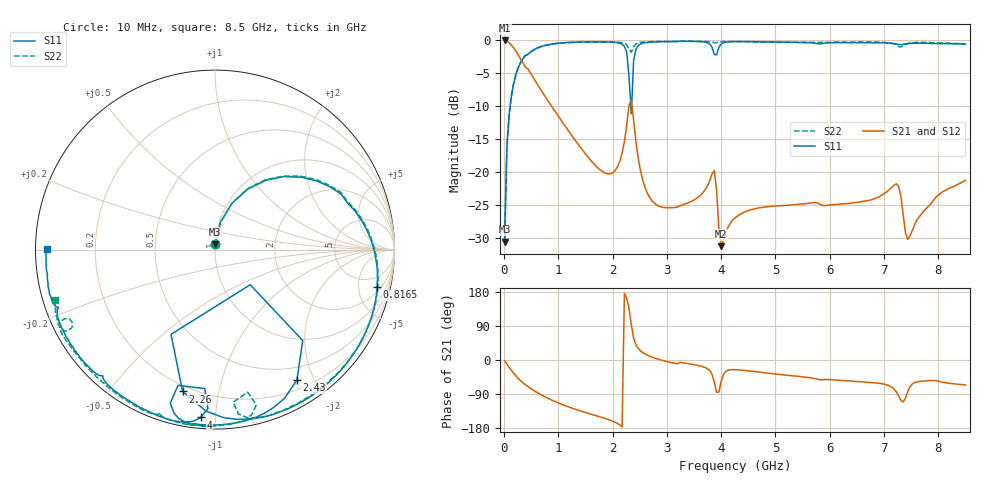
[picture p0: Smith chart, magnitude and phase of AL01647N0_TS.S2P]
!AVX CORPORATION
!PART NUMBER AL01647N0_TS
!DESCRIPTION: AIR CORE INDUCTOR, 47nH, 6 TURNS
!Agilent Technologies,E5071C,MY46102230,A.09.54
!Date: Mon Sep 03 16:36:54 2012
!Data & Calibration Information:
!Freq	S11:SOLT2(ON)	S21:SOLT2(ON)	S12:SOLT2(ON)	S22:SOLT2(ON)
# Hz S dB R 50
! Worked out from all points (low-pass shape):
!   201 points, 10 MHz to 8.5 GHz, reference 50 ohm
!   highest |S21| = -0.01 dB at 10 MHz (marker M1); lowest = -31.2 dB at 4 GHz (marker M2)
!   |S21| within 3 dB of the highest: start of sweep to 319.1 MHz
!   lowest |S11| = -30.5 dB at 10 MHz (marker M3), VSWR 1.06, Z = 50 + j2.98 ohm
!   |S11| at or under -10 dB: start of sweep to 112.4 MHz; 2.336 GHz to 2.351 GHz (14.6 MHz wide, 0.623 % of centre)
!   |S22| runs from -30.4 to -0.1 dB; largest |S21 - S12| = 0.0068
!   S11 on the Smith chart (normalised r, x): 10 MHz: 1.00, +0.06; 816.5 MHz: 2.65, -7.89; 2.26 GHz: 0.17, -0.78; 2.43 GHz: 0.32, -1.77; 4 GHz: 0.06, -0.92; 8.5 GHz: 0.03, +0.00
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1e7  -30.51 88.2  -0.01 -2.1  0.05 -2.1  -30.43 88.9
5.245e7  -16.06 78.5  -0.12 -11.1  -0.10 -11.2  -16.02 78.6
1.798e8  -6.42 53.8  -1.18 -35.6  -1.16 -35.6  -6.38 54.2
3.9205e8  -2.29 23.6  -4.05 -65.5  -4.02 -65.6  -2.26 24.3
8.1655e8  -0.65 -13.0  -9.26 -101.7  -9.26 -101.8  -0.64 -12.1
1.4533e9  -0.23 -48.5  -16.72 -136.5  -16.72 -136.5  -0.27 -47.7
2.00515e9  -0.26 -74.4  -20.06 -161.5  -20.06 -161.5  -0.25 -70.3
2.25985e9  -1.82 -102.9  -12.82 162.5  -12.82 162.5  -0.67 -81.9
2.3023e9  -5.48 -117.4  -9.82 136.8  -9.82 136.8  -1.36 -83.2
2.34475e9  -11.15 -44.9  -9.04 92.5  -9.03 92.4  -1.78 -77.1
2.3872e9  -3.05 -46.0  -12.07 57.5  -12.06 57.5  -0.96 -75.1
2.42965e9  -1.33 -57.8  -15.37 40.0  -15.36 40.0  -0.54 -77.3
2.85415e9  -0.22 -86.9  -25.14 1.5  -25.13 1.7  -0.16 -91.1
3.6607e9  -0.21 -99.5  -23.10 -17.5  -23.10 -17.6  -0.15 -104.5
3.87295e9  -2.11 -105.2  -19.76 -57.7  -19.77 -57.7  -0.36 -108.7
4.0003e9  -0.55 -94.9  -31.20 -55.6  -31.18 -55.8  -0.21 -110.2
4.255e9  -0.18 -102.6  -26.94 -25.6  -26.95 -25.8  -0.20 -115.7
5.6983e9  -0.39 -130.0  -24.60 -48.3  -24.64 -48.3  -0.30 -140.7
7.09915e9  -0.41 -156.7  -22.62 -68.4  -22.62 -68.3  -0.37 -154.4
7.26895e9  -0.60 -159.6  -22.11 -95.1  -22.12 -95.0  -0.93 -154.7
7.43875e9  -0.48 -161.1  -30.17 -83.3  -30.15 -83.0  -0.46 -151.4
8.5e9  -0.55 179.7  -21.21 -65.9  -21.23 -65.9  -0.59 -162.3
